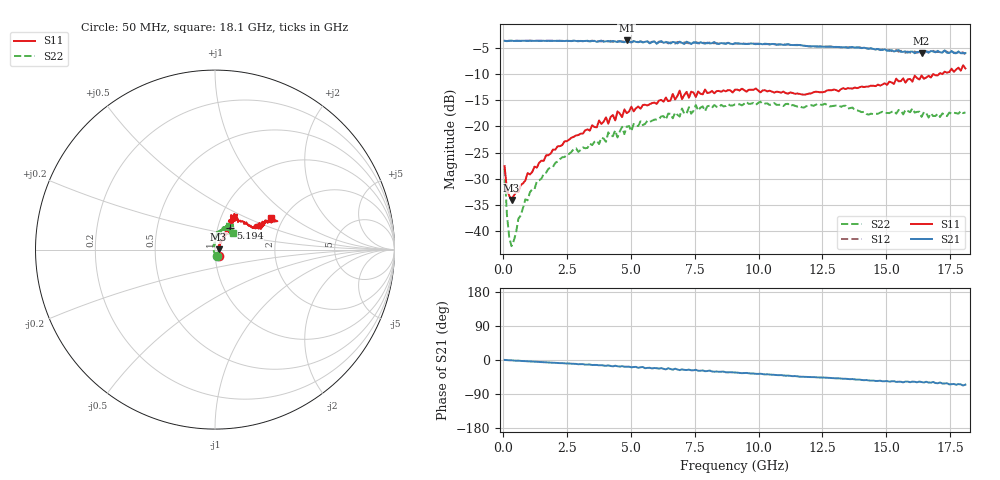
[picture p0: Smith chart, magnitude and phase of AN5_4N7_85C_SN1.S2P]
! Network Analyzer HP8720D.06.14 Serial No. US36140669
!  5 Jul 2005  07:06:41
! Frequency  S11  S21  S12  S22
# HZ  S  DB R 50
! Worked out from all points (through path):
!   201 points, 50 MHz to 18.1 GHz, reference 50 ohm
!   highest |S21| = -3.62 dB at 4.833 GHz (marker M1); lowest = -6.1 dB at 16.39 GHz (marker M2)
!   group delay of S21, straight-line fit = 10.2 ps
!   lowest |S11| = -34.0 dB at 320.8 MHz (marker M3), VSWR 1.04, Z = 52 + j0.156 ohm
!   |S11| at or under -10 dB: start of sweep to 17.08 GHz; 17.17908 GHz to 17.20526 GHz (26.18 MHz wide, 0.152 % of centre)
!   |S22| runs from -42.9 to -15.3 dB; largest |S21 - S12| = 0.031
!   S11 on the Smith chart (normalised r, x): 50 MHz: 1.05, -0.07; 5.194 GHz: 1.15, +0.29; 18.1 GHz: 1.73, +0.69
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5e7  -27.60 -53.4  -3.68 0.2  -3.70 0.5  -28.09 -77.0
1.4025e8  -32.05 -30.3  -3.76 -0.3  -3.71 -0.2  -36.87 -114.8
2.305e8  -33.23 -10.0  -3.68 -0.7  -3.68 -0.5  -41.15 -143.2
3.2075e8  -34.05 4.3  -3.65 -0.8  -3.68 -0.7  -42.87 178.1
8.6225e8  -30.32 38.7  -3.69 -2.8  -3.69 -2.9  -33.93 114.9
1.3135e9  -27.88 50.5  -3.67 -4.6  -3.69 -4.5  -30.48 95.2
3.1185e9  -21.37 56.7  -3.74 -10.8  -3.77 -11.2  -24.03 88.8
4.021e9  -18.29 58.2  -3.78 -15.3  -3.80 -14.2  -22.97 82.1
4.382e9  -18.86 57.4  -3.81 -15.2  -3.81 -16.4  -20.78 82.3
4.47225e9  -17.15 54.3  -3.92 -16.5  -3.74 -15.7  -22.13 84.9
4.83325e9  -17.48 63.0  -3.62 -17.7  -3.81 -18.1  -20.06 72.8
5.19425e9  -16.56 55.1  -3.89 -18.2  -3.77 -18.5  -19.93 80.6
6.09675e9  -15.09 58.5  -3.93 -22.9  -3.83 -22.4  -18.59 69.7
6.7285e9  -14.88 64.3  -3.97 -23.0  -4.23 -23.8  -17.39 62.7
6.909e9  -13.19 61.0  -3.84 -26.7  -3.94 -24.9  -18.13 62.7
6.99925e9  -14.79 61.0  -4.09 -24.7  -4.25 -26.5  -16.61 63.6
9.075e9  -13.00 59.5  -4.18 -33.0  -4.16 -33.0  -15.82 55.5
1.21435e10  -13.52 49.3  -4.73 -45.1  -4.69 -45.1  -16.10 63.1
1.512175e10  -11.47 27.8  -5.60 -57.1  -5.42 -56.4  -17.48 56.9
1.602425e10  -11.47 27.6  -5.73 -56.9  -5.99 -59.0  -16.58 47.0
1.638525e10  -10.31 27.0  -6.07 -58.1  -5.79 -57.4  -18.19 45.3
1.81e10  -8.95 29.3  -6.01 -65.0  -6.28 -65.7  -17.35 41.7
